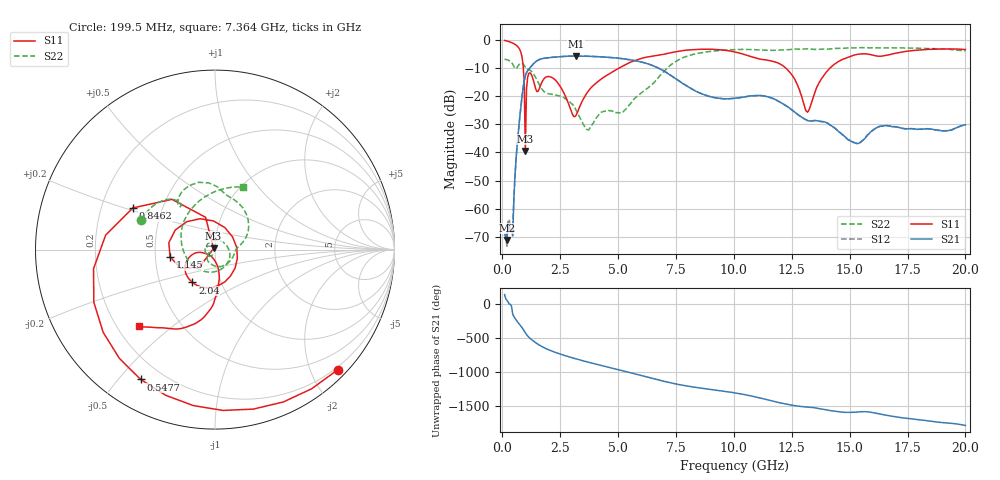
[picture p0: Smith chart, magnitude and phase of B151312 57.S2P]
!  2-Port S-parameters saved by WinCal
! VAR MeasName=S-Parameters (CALIBRATED_DATA) read from VNA (N5244A)
! VAR MeasDate=12/8/2015 5:48:15 PM
! VAR NAME=B151312 57
! VAR FILENAME=B151312 57.S2P
! VAR DATE=12/8/2015 5:48:15 PM
! VAR PHYS_PORTS=1,2
# Hz S DB R 50
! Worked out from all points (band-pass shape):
!   401 points, 100 MHz to 20 GHz, reference 50 ohm
!   highest |S21| = -5.74 dB at 3.184 GHz (marker M1); lowest = -71.1 dB at 199.5 MHz (marker M2)
!   |S21| within 3 dB of the highest: 1.319 GHz to 6.366 GHz (5.047 GHz wide, 131 % of centre)
!   lowest |S11| = -39.5 dB at 995.5 MHz (marker M3), VSWR 1.02, Z = 49.2 + j0.691 ohm
!   |S11| at or under -10 dB: 907.3 MHz to 5.046 GHz (4.139 GHz wide, 139 % of centre); 12.24 GHz to 14.15 GHz (1.915 GHz wide, 14.5 % of centre)
!   |S22| runs from -32.0 to -2.7 dB; largest |S21 - S12| = 0.0019
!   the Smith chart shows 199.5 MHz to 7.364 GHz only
!   S11 on the Smith chart (normalised r, x): 199.5 MHz: 0.15, -2.44; 547.8 MHz: 0.12, -0.57; 846.2 MHz: 0.34, +0.21; 1.145 GHz: 0.60, -0.05; 2.04 GHz: 0.73, -0.28; 7.364 GHz: 0.29, -0.39
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1e8  -0.20 -22.6  -69.40 135.1  -70.54 129.7  -6.89 169.3
1.995e8  -0.38 -44.4  -71.11 50.4  -73.35 52.5  -7.05 158.3
3.985e8  -0.94 -87.2  -67.14 -36.4  -67.97 -48.5  -8.06 135.5
5.4775e8  -1.58 -119.8  -48.51 145.1  -48.45 145.3  -10.12 126.7
8.4625e8  -5.80 153.1  -20.58 10.1  -20.58 10.0  -8.28 103.7
9.955e8  -39.53 138.3  -12.79 -68.4  -12.79 -68.5  -9.69 83.0
1.14475e9  -11.93 -170.5  -10.42 -132.4  -10.42 -132.4  -10.53 68.8
1.64225e9  -16.37 -42.4  -6.86 101.7  -6.86 101.7  -16.57 11.7
2.04025e9  -13.06 -124.5  -6.29 35.8  -6.28 35.7  -19.18 -13.4
3.1845e9  -26.82 -110.1  -5.74 -92.7  -5.74 -92.7  -25.00 -138.6
3.43325e9  -22.09 -83.9  -5.76 -116.1  -5.76 -116.1  -28.84 -152.8
4.22925e9  -14.17 -84.5  -6.00 173.7  -6.00 173.6  -26.14 -131.6
5.075e9  -9.87 -93.2  -6.56 101.9  -6.56 102.0  -25.84 104.2
5.9705e9  -6.66 -111.0  -7.79 25.3  -7.77 25.1  -19.06 -66.3
6.7665e9  -5.41 -125.6  -10.12 -44.6  -10.11 -44.6  -13.10 146.2
7.3635e9  -4.41 -134.8  -13.07 -92.7  -13.06 -92.9  -8.36 65.7
8.3585e9  -3.38 -155.1  -18.25 -153.0  -18.22 -153.4  -4.92 -8.3
1.005e10  -4.30 168.9  -20.74 125.7  -20.75 125.3  -3.43 -69.8
1.338325e10  -21.42 -54.3  -28.85 -88.5  -28.86 -88.3  -3.32 -120.8
1.45275e10  -7.63 -115.1  -32.59 -152.7  -32.55 -153.0  -3.04 -130.5
1.67165e10  -5.27 -155.5  -30.67 147.7  -30.57 147.4  -2.80 -152.3
2e10  -3.44 161.7  -30.17 6.2  -30.33 5.7  -3.90 -179.9
